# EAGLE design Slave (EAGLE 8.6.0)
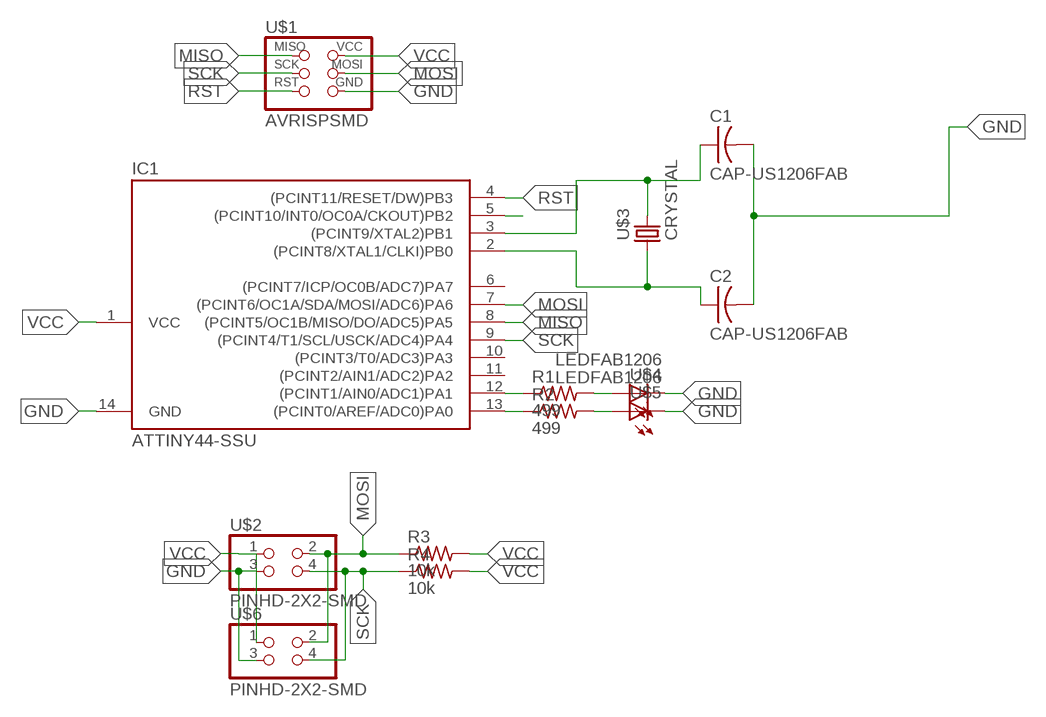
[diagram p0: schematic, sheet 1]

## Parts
C1  CAP-US1206FAB  [C1206FAB]
C2  CAP-US1206FAB  [C1206FAB]
IC1  ATTINY44-SSU  [SOIC14]
R1  499  RES-US1206FAB  [R1206FAB]
R2  499  RES-US1206FAB  [R1206FAB]
R3  10k  RES-US1206FAB  [R1206FAB]
R4  10k  RES-US1206FAB  [R1206FAB]
U$1  AVRISPSMD  [2X03SMD]
U$2  PINHD-2X2-SMD  [2X02SMD]
U$3  CRYSTAL  [2-SMD-5X3MM]
U$4  LEDFAB1206  [LED1206FAB]
U$5  LEDFAB1206  [LED1206FAB]
U$6  PINHD-2X2-SMD  [2X02SMD]

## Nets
GND: C1.2 C2.2 IC1.14(GND) U$1.6(GND) U$2.3 U$4.2(C) U$5.2(C) U$6.3
MISO: IC1.8((PCINT5/OC1B/MISO/DO/ADC5)PA5) U$1.1(MISO)
MOSI: IC1.7((PCINT6/OC1A/SDA/MOSI/ADC6)PA6) R3.1 U$1.4(MOSI) U$2.2 U$6.2
N$1: IC1.12((PCINT1/AIN0/ADC1)PA1) R1.1
N$2: IC1.13((PCINT0/AREF/ADC0)PA0) R2.1
N$3: R1.2 U$4.1(A)
N$4: R2.2 U$5.1(A)
N$10: IC1.5((PCINT10/INT0/OC0A/CKOUT)PB2)
N$11: C1.1 IC1.3((PCINT9/XTAL2)PB1) U$3.P$2
N$12: C2.1 IC1.2((PCINT8/XTAL1/CLKI)PB0) U$3.P$1
RST: IC1.4((PCINT11/RESET/DW)PB3) U$1.5(RST)
SCK: IC1.9((PCINT4/T1/SCL/USCK/ADC4)PA4) R4.1 U$1.3(SCK) U$2.4 U$6.4
VCC: IC1.1(VCC) R3.2 R4.2 U$1.2(VCC) U$2.1 U$6.1
Unconnected: IC1.6((PCINT7/ICP/OC0B/ADC7)PA7) IC1.10((PCINT3/T0/ADC3)PA3) IC1.11((PCINT2/AIN1/ADC2)PA2)

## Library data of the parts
C1 C2 = fab:CAP-US
IC1 = fab:ATTINY44
R1-R4 = fab:RES-US: Resistor (US Symbol)
U$1 = fab:AVRISP
U$2 U$6 = fab:PINHD-2X2-SMD
U$3 = fab:CRYSTAL
U$4 U$5 = fab:LED: LED

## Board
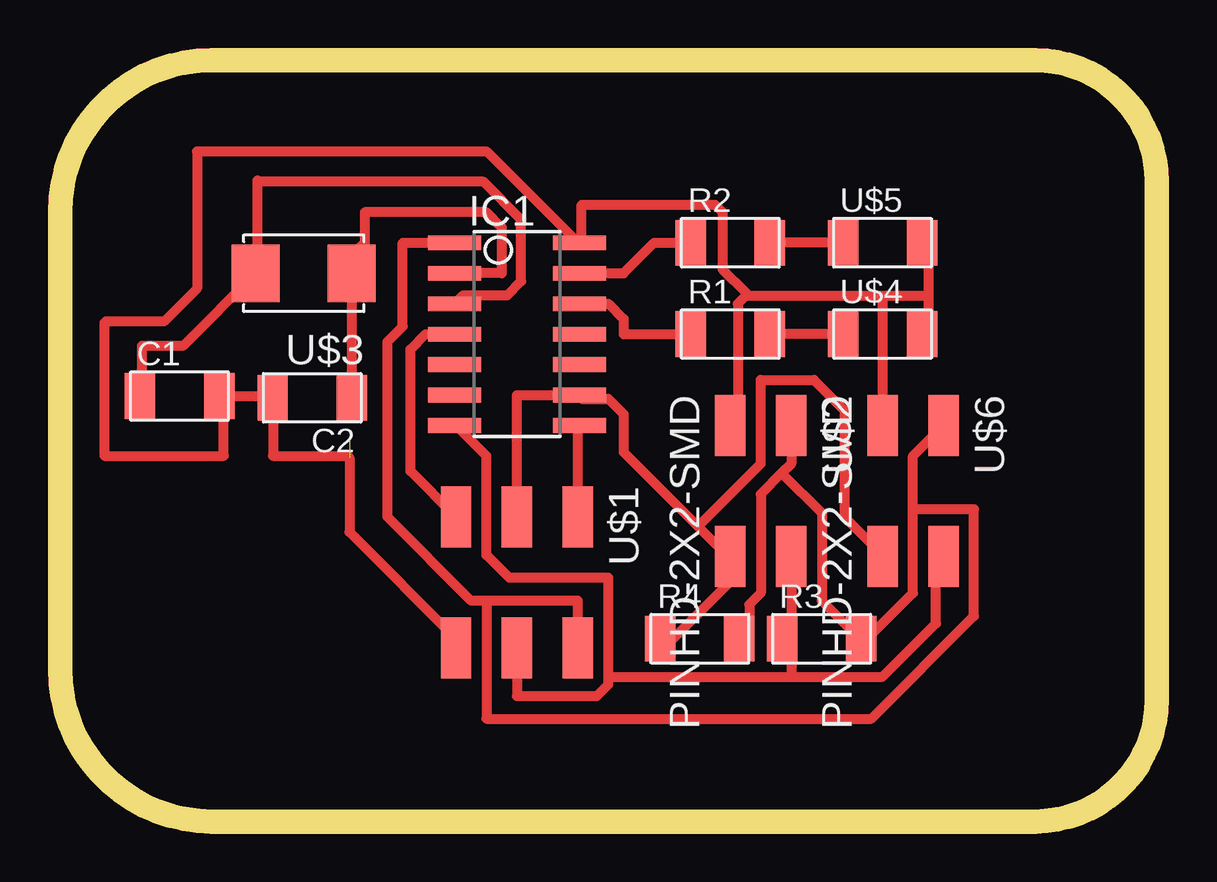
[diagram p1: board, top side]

Size 45.72 x 31.75 mm. Coordinates in mm from the lower left corner, seen from the top.
Outline: 0,25.4 0,6.35 arc90 6.35,0 40.64,0 arc90 45.72,5.08 45.72,26.67 arc90 40.64,31.75 6.35,31.75 arc90 0,25.4
Copper layers (1*16): Top 0.035mm / dielectric 1.5mm / Bottom 0.035mm
Design rules "default *": minimum track width 16mil, minimum drill 0.35mm, track to track 16mil, track to pad 16mil, pad to pad 16mil, via to via 16mil, smd to smd 16mil, copper to edge 16mil, drill to drill 16mil, minimum pad ring 10mil, minimum via ring 8mil, stop-mask expansion 4mil, vias tented up to drill 0mil, thermal gap 10mil

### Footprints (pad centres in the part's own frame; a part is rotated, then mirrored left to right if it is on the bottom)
C1206FAB = smd 1.27 x 1.905: 1 -1.651,0; 2 1.651,0
SOIC14 = smd 0.61 x 2.21: 1 -3.81,-2.603; 2 -2.54,-2.603; 3 -1.27,-2.603; 4 0,-2.603; 5 1.27,-2.603; 6 2.54,-2.603; 7 3.81,-2.603; 8 3.81,2.603; 9 2.54,2.603; 10 1.27,2.603; 11 0,2.603; 12 -1.27,2.603; 13 -2.54,2.603; 14 -3.81,2.603
R1206FAB = smd 1.27 x 1.905: 1 -1.651,0; 2 1.651,0
2X03SMD = smd 2.54 x 1.27: 1 -2.54,2.54; 2 2.92,2.54; 3 -2.54,0; 4 2.92,0; 5 -2.54,-2.54; 6 2.92,-2.54
2X02SMD = smd 2.54 x 1.27: 1 -2.54,1.27; 2 2.92,1.27; 3 -2.54,-1.27; 4 2.92,-1.27
2-SMD-5X3MM = smd 2 x 2.4: P$1 -2,0; P$2 2,0
LED1206FAB = smd 1.27 x 1.905: 1 -1.651,0; 2 1.651,0

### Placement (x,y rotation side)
C1  4.99,17.74 0 top
C2  10.52,17.67 180 top
IC1  19.05,20.32 270 top
R1  27.94,20.32 0 top
R2  27.94,24.13 0 top
R3  31.75,7.62 0 top
R4  26.67,7.62 0 top
U$1  19.05,10.16 270 top
U$2  29.21,13.97 270 top
U$3  10.16,22.86 180 top
U$4  34.29,20.32 0 top
U$5  34.29,24.13 0 top
U$6  35.56,13.97 270 top

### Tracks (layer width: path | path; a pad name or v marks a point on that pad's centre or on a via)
GND  (1 unrouted)
  Top 0.406: 36.2,21.91 36.2,24.13 U$5.2 | 36.2,21.91 36.2,20.32 U$4.2 | U$1.6 16.51,7.62 12.06,12.07 12.06,15.18 12,15.24 8.88,15.24 8.88,17.65 C2.2 8.25,17.74 6.9,17.74 | U$2.3 28.26,16.83 28.26,21.59 28.57,21.91 | 36.2,21.91 34.29,21.91 | 34.29,21.91 28.57,21.91 | 34.29,21.91 U$6.3 | 28.57,21.91 28.57,22.07 27.62,23.02 27.62,25.4 27.3,25.72 21.75,25.72 21.75,24.29 IC1.14 21.59,24.13 17.78,27.94 5.71,27.94 5.71,22.23 4.34,20.85 1.91,20.85 1.84,20.78 1.84,15.24 6.83,15.24 6.83,17.67 6.9,17.74 | C1.2 6.9,17.74
MISO
  Top 0.406: U$1.1 21.59,16.51 IC1.8
MOSI
  Top 0.406: 30.48,7.62 R3.1 | U$2.2 30.48,7.78 R3.1 | 30.48,6.03 34.29,6.03 36.51,8.25 36.51,10.64 36.83,10.95 U$6.2 | 30.48,6.03 30.48,7.46 R3.1 | 22.86,6.03 22.86,5.72 22.38,5.24 19.05,5.24 U$1.4 | 22.86,6.03 22.86,10.16 18.73,10.16 17.78,11.11 17.78,15.24 16.51,16.51 IC1.7 | 22.86,6.03 30.48,6.03
N$1
  Top 0.406: R1.1 23.5,20.32 23.5,20.96 22.86,21.59 IC1.12
N$2
  Top 0.406: R2.1 24.77,24.13 23.5,22.86 IC1.13
N$3
  Top 0.406: U$4.1 R1.2
N$4
  Top 0.406: U$5.1 R2.2
N$11
  Top 0.406: IC1.3 16.8,21.95 18.65,21.95 19.23,22.52 19.23,25.1 17.66,26.67 8.28,26.67 8.22,26.73 8.22,22.92 U$3.P$2 5.13,19.83 3.42,19.83 3.42,18.25 3.34,18.17 C1.1
N$12
  Top 0.406: IC1.2 18.41,22.86 18.41,24.77 17.78,25.4 12.7,25.4 12.7,24.13 12.16,23.59 U$3.P$1 C2.1
RST
  Top 0.406: IC1.4 15.24,20.32 14.61,19.69 14.61,14.61 U$1.5
SCK
  Top 0.406: U$2.4 27.94,10.16 | 25.4,7.62 R4.1 | U$1.3 19.05,17.78 IC1.9 21.75,17.62 22.86,17.62 23.5,16.99 23.5,15.4 26.59,12.3 | 24.77,7.62 R4.1 | R4.1 25.56,7.62 27.94,10 U$2.4 | 26.59,12.3 27.78,11.11 U$2.4 | 26.59,12.3 29.21,14.92 29.21,18.41 31.43,18.41 32.7,17.14 32.7,12.7 34.29,11.11 U$6.4
VCC
  Top 0.406: 27.94,7.62 R4.2 28.42,7.78 28.73,8.1 28.73,9.05 29.21,9.52 29.21,13.65 30.08,14.53 | 30.08,14.53 30.48,14.92 U$2.1 | 30.08,14.53 31.75,12.86 31.75,9.21 33.34,7.62 R3.2 33.5,7.46 35.56,9.52 35.56,13.02 | U$6.1 35.56,15.24 35.56,13.02 | IC1.1 14.29,24.13 14.29,20.64 13.65,20 13.65,12.7 17.14,9.21 17.78,9.21 | 17.78,9.21 21.59,9.21 U$1.2 | 35.56,13.02 38.1,13.02 38.1,8.57 33.81,4.29 17.78,4.29 17.78,9.21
